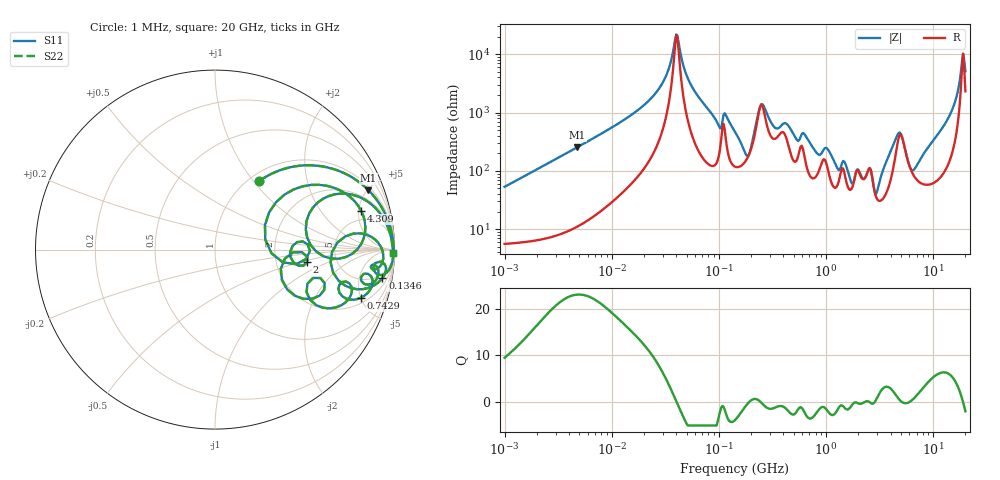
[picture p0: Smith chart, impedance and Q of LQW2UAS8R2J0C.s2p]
!Murata Part Number: LQW2UAS8R2J0C
!These Parameters are Measured in Series Mode Connection
!  o--[Z]--o
!Port1  Port2
!  o-------o
!Freq. Start=1[MHz] Stop=20[GHz], 401[Steps]
# Hz S RI R 50
!Freq.(Hz) S11(Real) S11(Imag) S21(Real) S21(Imag) S12(Real) S12(Imag) S22(Real) S22(Imag)
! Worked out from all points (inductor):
!   401 points, 1 MHz to 20 GHz, reference 50 ohm
!   read as one part in series: L = 8.42 uH near 1.051 MHz
!   highest Q = 23 at 4.758 MHz (marker M1), where L = 8.48 uH
!   self-resonance near 40.01 MHz
!   S11 on the Smith chart (normalised r, x): 1 MHz: 1.11, +1.06; 134.6 MHz: 4, -11; 742.9 MHz: 2.50, -5.02; 2 GHz: 3.03, -0.59; 4.309 GHz: 3.59, +5.34; 20 GHz: open
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1000000  0.2438 0.38  0.7562 -0.38  0.7562 -0.38  0.2438 0.38
4757866  0.8551 0.331  0.1449 -0.331  0.1449 -0.331  0.8551 0.331
5253183  0.8771 0.3073  0.1229 -0.3073  0.1229 -0.3073  0.8771 0.3073
2.759593e7  0.9936 0.0382  0.00642 -0.0382  0.00642 -0.0382  0.9936 0.0382
4.100967e7  0.9955 -0.00164  0.00448 0.00164  0.00448 0.00164  0.9955 -0.00164
5.945315e7  0.9926 -0.0422  0.00743 0.0422  0.00743 0.0422  0.9926 -0.0422
1.345891e8  0.9323 -0.1591  0.0677 0.1591  0.0677 0.1591  0.9323 -0.1591
1.414214e8  0.9143 -0.1788  0.0857 0.1788  0.0857 0.1788  0.9143 -0.1788
1.856921e8  0.6442 -0.0722  0.3558 0.0722  0.3558 0.0722  0.6442 -0.0722
2.561986e8  0.9368 -0.0244  0.0632 0.0244  0.0632 0.0244  0.9368 -0.0244
3.281728e8  0.8873 -0.1103  0.1127 0.1103  0.1127 0.1103  0.8873 -0.1103
7.429123e8  0.8132 -0.2682  0.1868 0.2682  0.1868 0.2682  0.8132 -0.2682
2.000048e9  0.5135 -0.071  0.4865 0.071  0.4865 0.071  0.5135 -0.071
2.972225e9  0.2783 0.1359  0.7217 -0.1359  0.7217 -0.1359  0.2783 0.1359
3.902654e9  0.7274 0.3126  0.2726 -0.3126  0.2726 -0.3126  0.7274 0.3126
4.308939e9  0.815 0.2155  0.185 -0.2155  0.185 -0.2155  0.815 0.2155
4.999031e9  0.8139 0.0302  0.1861 -0.0302  0.1861 -0.0302  0.8139 0.0302
6.403413e9  0.5056 0.1156  0.4944 -0.1156  0.4944 -0.1156  0.5056 0.1156
8.834765e9  0.8046 0.2927  0.1954 -0.2927  0.1954 -0.2927  0.8046 0.2927
1.449594e10  0.9724 0.0986  0.0276 -0.0986  0.0276 -0.0986  0.9724 0.0986
1.856831e10  0.9897 0.00879  0.0103 -0.00879  0.0103 -0.00879  0.9897 0.00879
2e10  0.9909 -0.0172  0.00911 0.0172  0.00911 0.0172  0.9909 -0.0172
